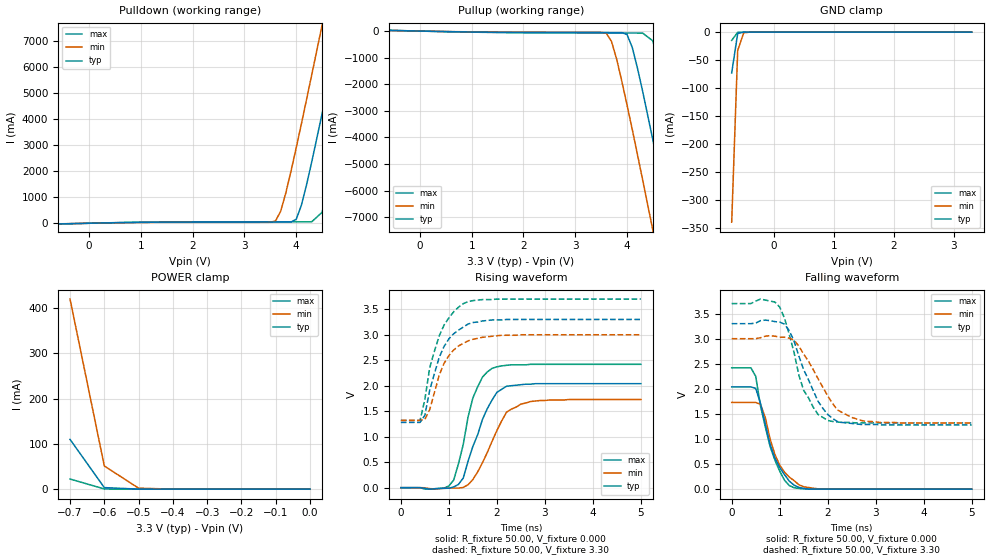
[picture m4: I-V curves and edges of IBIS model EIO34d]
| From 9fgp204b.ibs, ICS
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|   Model EIO34d
[Model]   EIO34d
Model_type   I/O
Polarity   Non-Inverting
Enable   Active-High
Vinl =   0.80V
Vinh =   2.00V
Vmeas =   1.50V
C_comp   3.40pF   2.85pF   3.95pF
[Temperature Range]   27.00   70.00   0.000
[Voltage Range]   3.30V   3.00V   3.70V
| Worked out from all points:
|   slope of the pulldown table from 0 to 0.495 V, typ, clamps not added: 24.5 ohm
|   slope of the pullup table from 0 to 0.495 V, typ, clamps not added: 25.6 ohm
|   GND clamp passes 1 mA (typ) near -0.54 V on its own axis
|   POWER clamp passes 1 mA (typ) near -0.53 V on its own axis
|   rising waveform, R_fixture 50.00, V_fixture 0.000: 20-80 % time 482ps typ, 523ps min, 376ps max; typ from 0 V to 2.04 V
|   rising waveform, R_fixture 50.00, V_fixture 3.30: 20-80 % time 430ps typ, 430ps min, 414ps max; typ from 1.28 V to 3.3 V
|   falling waveform, R_fixture 50.00, V_fixture 0.000: 20-80 % time 396ps typ, 385ps min, 390ps max; typ from 2.04 V to 0 V
|   falling waveform, R_fixture 50.00, V_fixture 3.30: 20-80 % time 529ps typ, 623ps min, 456ps max; typ from 3.3 V to 1.28 V
[Pulldown]
| voltage   I(typ)   I(min)   I(max)
|  -3.30   0.000A   -0.13A   10.00mA
|  -3.10   0.000A   0.000A   0.000A
|  -2.90   0.000A   0.000A   0.000A
|  -2.70   0.000A   0.000A   0.000A
|  -2.50   0.000A   0.000A   0.000A
|  -2.30   0.000A   0.000A   0.000A
|  -2.10   0.000A   0.000A   0.000A
|  -1.90   0.000A   0.000A   0.000A
|  -1.70   -1.00mA   -1.00mA   -1.00mA
|  -1.50   -2.00mA   -1.00mA   -1.00mA
|  -1.00   -4.00mA   -3.00mA   -4.00mA
|  -0.90   -5.00mA   -4.00mA   -7.00mA
|  -0.80   -10.10mA   -6.00mA   -15.50mA
|  -0.70   -23.05mA   -11.80mA   -30.08mA
-600mV    -25.74mA   -20.62mA   -28.02mA
3.6V      45.68mA    87.67mA    56.32mA
3.7V      45.72mA    460mA      56.36mA
4V        150mA      2.9A       56.49mA
4.1V      690mA      3.82A      56.55mA
4.3V      2.36A      5.71A      57.08mA
4.5V      4.21A      7.62A      420mA
4.7V      6.12A      9.56A      2.03A
4.9V      8.05A      11.51A     3.88A
5.1V      10A        13.46A     5.79A
5.3V      11.95A     15.43A     7.72A
6.6V      24.8A      28.28A     20.52A
[Pullup]
| voltage   I(typ)   I(min)   I(max)
|  -3.30   0.000A   0.000A   0.000A
|  -3.10   0.000A   10.00mA   0.000A
|  -2.90   10.00mA   0.000A   0.000A
|  -2.70   0.000A   0.000A   0.000A
|  -2.50   0.000A   0.000A   0.000A
|  -2.30   0.000A   0.000A   0.000A
|  -2.10   0.000A   0.000A   0.000A
|  -1.90   0.000A   0.000A   0.000A
|  -1.70   1.00mA   1.00mA   1.00mA
|  -1.50   2.00mA   1.00mA   1.00mA
|  -1.00   4.00mA   3.00mA   4.00mA
|  -0.90   5.00mA   3.00mA   7.00mA
|  -0.80   9.70mA   6.00mA   14.90mA
|  -0.70   22.10mA   11.00mA   31.25mA
-600mV    26.38mA    20.34mA    29.23mA
3.6V      -57.31mA   -78.9mA    -72.07mA
3.7V      -57.52mA   -390mA     -72.33mA
3.8V      -57.8mA    -1.06A     -72.58mA
4V        -130mA     -2.78A     -73.05mA
4.1V      -610mA     -3.69A     -73.27mA
4.3V      -2.25A     -5.58A     -74.12mA
4.5V      -4.1A      -7.5A      -370mA
4.7V      -6.01A     -9.43A     -1.94A
4.9V      -7.94A     -11.38A    -3.78A
5.3V      -11.85A    -15.31A    -7.63A
6.6V      -24.71A    -28.18A    -20.45A
[GND_clamp]
| voltage   I(typ)   I(min)   I(max)
|  -3.30   -24.57A   -25.08A   -24.27A
|  -3.20   -23.58A   -24.09A   -23.27A
|  -3.10   -22.59A   -23.10A   -22.28A
|  -3.00   -21.60A   -22.11A   -21.29A
|  -2.90   -20.61A   -21.12A   -20.30A
|  -2.80   -19.63A   -20.13A   -19.31A
|  -2.70   -18.64A   -19.15A   -18.33A
|  -2.60   -17.65A   -18.16A   -17.34A
|  -2.50   -16.67A   -17.18A   -16.35A
|  -2.40   -15.68A   -16.20A   -15.36A
|  -2.30   -14.70A   -15.21A   -14.38A
|  -2.20   -13.72A   -14.23A   -13.40A
|  -2.10   -12.73A   -13.25A   -12.41A
|  -2.00   -11.75A   -12.28A   -11.43A
|  -1.90   -10.78A   -11.30A   -10.45A
|  -1.80   -9.80A   -10.33A   -9.48A
|  -1.70   -8.83A   -9.36A   -8.50A
|  -1.60   -7.86A   -8.39A   -7.53A
|  -1.50   -6.89A   -7.43A   -6.56A
|  -1.40   -5.93A   -6.47A   -5.60A
|  -1.30   -4.98A   -5.51A   -4.64A
|  -1.20   -4.03A   -4.57A   -3.70A
|  -1.10   -3.10A   -3.64A   -2.77A
|  -1.00   -2.19A   -2.72A   -1.86A
|  -0.90   -1.32A   -1.84A   -1.00A
|  -0.80   -0.55A   -1.01A   -0.29A
-700mV    -72.95mA   -340mA     -14.76mA
-600mV    -2.33mA    -32.82mA   -460uA
-500mV    -100uA     -1.33mA    -46.85uA
-300mV    -9.64uA    -9.52uA    -11.49uA
3.3V      35.65uA    26.86uA    51.23uA
[POWER_clamp]
| voltage   I(typ)   I(min)   I(max)
|  -3.30   24.70A   25.22A   24.38A
|  -3.20   23.71A   24.23A   23.39A
|  -3.10   22.72A   23.24A   22.40A
|  -3.00   21.73A   22.26A   21.41A
|  -2.90   20.74A   21.27A   20.42A
|  -2.80   19.76A   20.28A   19.43A
|  -2.70   18.77A   19.30A   18.44A
|  -2.60   17.78A   18.31A   17.46A
|  -2.50   16.80A   17.33A   16.47A
|  -2.40   15.81A   16.34A   15.48A
|  -2.30   14.83A   15.36A   14.50A
|  -2.20   13.84A   14.38A   13.51A
|  -2.10   12.86A   13.40A   12.53A
|  -2.00   11.88A   12.42A   11.55A
|  -1.90   10.90A   11.45A   10.57A
|  -1.80   9.93A   10.47A   9.60A
|  -1.70   8.96A   9.51A   8.62A
|  -1.60   7.99A   8.54A   7.65A
|  -1.50   7.02A   7.57A   6.68A
|  -1.40   6.06A   6.61A   5.72A
|  -1.30   5.10A   5.66A   4.76A
|  -1.20   4.16A   4.71A   3.81A
|  -1.10   3.22A   3.78A   2.88A
|  -1.00   2.31A   2.86A   1.97A
|  -0.90   1.43A   1.97A   1.10A
|  -0.80   0.64A   1.13A   0.36A
-700mV    110mA      420mA      22.45mA
-600mV    3.45mA     51.17mA    440uA
-500mV    120uA      2.16mA     57.35uA
-400mV    37.43uA    100uA      51.38uA
-300mV    35.71uA    26.86uA    51.29uA
-200mV    35.67uA    24.17uA    51.28uA
-100mV    35.66uA    24.07uA    51.27uA
0V        35.65nA    24.07nA    51.27nA
[Ramp]
| variable   typ   min   max
dV/dt_r   1.22/0.46n   1.04/0.55n   1.45/0.37n
dV/dt_f   1.21/0.52n   1.01/0.64n   1.43/0.45n
R_load = 50.00
[Rising Waveform]
R_fixture = 50.00
V_fixture = 0.000
V_fixture_min = 0.000
V_fixture_max = 0.000
| time   V(typ)   V(min)   V(max)
0s        390uV      300uV      480uV
900ps     -11.44mV   -12.82mV   -8.34mV
1.1ns     14.41mV    -8.26mV    150mV
1.3ns     190mV      5.18mV     850mV
1.5ns     810mV      160mV      1.76V
1.7ns     1.34V      490mV      2.17V
1.9ns     1.72V      910mV      2.34V
2.2ns     1.99V      1.48V      2.4V
2.5ns     2.02V      1.64V      2.41V
5ns       2.04V      1.73V      2.42V
[Rising Waveform]
R_fixture = 50.00
V_fixture = 3.30
V_fixture_min = 3.00
V_fixture_max = 3.70
| time   V(typ)   V(min)   V(max)
0s        1.28V      1.32V      1.32V
400ps     1.28V      1.32V      1.32V
500ps     1.42V      1.34V      1.73V
600ps     1.91V      1.53V      2.35V
800ps     2.56V      2.21V      2.98V
1ns       2.92V      2.59V      3.33V
1.3ns     3.15V      2.83V      3.61V
1.5ns     3.24V      2.91V      3.67V
2.1ns     3.29V      2.99V      3.7V
5ns       3.3V       3V         3.7V
[Falling Waveform]
R_fixture = 50.00
V_fixture = 0.000
V_fixture_min = 0.000
V_fixture_max = 0.000
| time   V(typ)   V(min)   V(max)
0s        2.04V      1.73V      2.42V
400ps     2.04V      1.73V      2.42V
500ps     2.01V      1.73V      2.25V
600ps     1.71V      1.69V      1.66V
700ps     1.3V       1.43V      1.24V
800ps     890mV      1V         850mV
1ns       430mV      480mV      360mV
1.2ns     160mV      240mV      71.84mV
1.8ns     2.38mV     6.44mV     1.64mV
5ns       430uV      350uV      580uV
[Falling Waveform]
R_fixture = 50.00
V_fixture = 3.30
V_fixture_min = 3.00
V_fixture_max = 3.70
| time   V(typ)   V(min)   V(max)
0s        3.3V       3V         3.7V
600ps     3.36V      3.02V      3.79V
1ns       3.33V      3.03V      3.63V
1.2ns     3.16V      3.01V      3.08V
1.5ns     2.38V      2.69V      1.97V
1.8ns     1.75V      2.2V       1.49V
2ns       1.49V      1.86V      1.37V
2.2ns     1.35V      1.58V      1.34V
2.8ns     1.29V      1.35V      1.32V
5ns       1.28V      1.32V      1.32V
